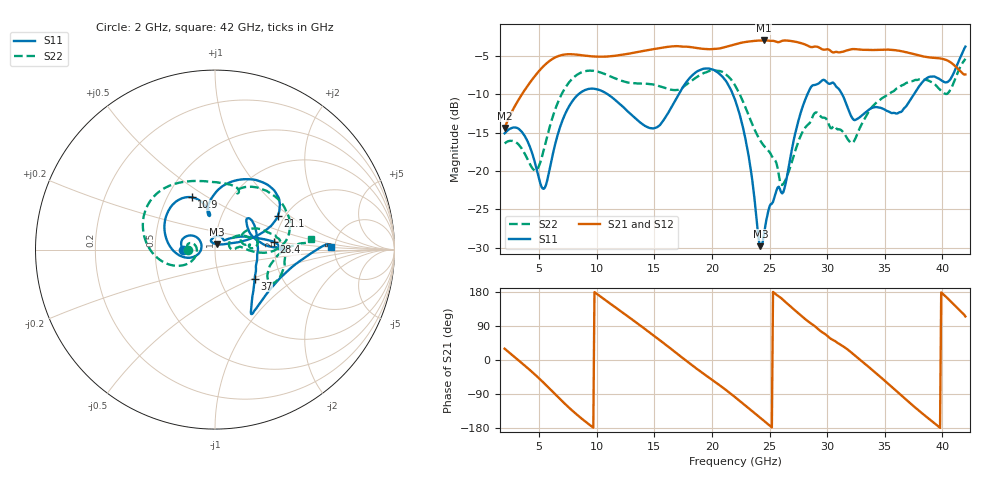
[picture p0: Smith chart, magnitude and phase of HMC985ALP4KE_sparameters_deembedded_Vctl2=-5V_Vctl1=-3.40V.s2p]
!s2p File: Measurements: S11, S21, S12, S22
# GHz S dB R 50.0
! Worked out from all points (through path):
!   401 points, 2 GHz to 42 GHz, reference 50 ohm
!   highest |S21| = -2.97 dB at 24.5 GHz (marker M1); lowest = -14.4 dB at 2 GHz (marker M2)
!   lowest |S11| = -29.8 dB at 24.2 GHz (marker M3), VSWR 1.07, Z = 50.8 + j3.16 ohm
!   |S11| at or under -10 dB: start of sweep to 8.403 GHz; 10.97 GHz to 17.11 GHz (6.144 GHz wide, 43.8 % of centre); 21.81 GHz to 28.29 GHz (6.471 GHz wide, 25.8 % of centre)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
!   |S22| runs from -21.8 to -5.4 dB; largest |S21 - S12| = 0.00075
!   S11 on the Smith chart (normalised r, x): 2 GHz: 0.70, -0.00; 10.9 GHz: 0.66, +0.43; 21.1 GHz: 1.84, +0.81; 28.4 GHz: 1.96, +0.19; 37 GHz: 1.46, -0.51; 42 GHz: 4.67, +0.19
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2  -15.08 -178.9  -14.38 29.8  -14.39 29.8  -16.39 -179.5
3.6  -15.10 155.1  -9.77 -10.9  -9.78 -10.9  -17.35 164.5
5.4  -22.31 174.3  -6.29 -60.3  -6.30 -60.3  -17.23 -154.6
6.9  -13.88 -171.0  -4.90 -105.7  -4.90 -105.7  -10.12 -169.4
8.7  -9.66 146.2  -4.90 -154.9  -4.90 -154.9  -7.12 153.5
10.9  -9.94 113.9  -5.07 154.7  -5.07 154.7  -7.47 118.4
13.4  -13.17 99.2  -4.52 99.5  -4.52 99.5  -8.55 84.5
15.4  -14.11 101.1  -3.99 53.9  -3.99 53.9  -8.92 68.5
17.9  -8.16 76.0  -3.80 -5.0  -3.80 -5.0  -8.60 67.0
21.1  -8.04 28.1  -3.85 -76.5  -3.86 -76.4  -7.27 15.7
22  -10.69 20.3  -3.48 -97.9  -3.48 -97.9  -8.82 2.1
23.1  -17.33 17.6  -3.13 -125.2  -3.13 -125.1  -12.41 -3.7
24.2  -29.78 73.2  -2.98 -152.5  -2.98 -152.5  -16.04 3.5
24.5  -28.34 106.3  -2.97 -160.1  -2.97 -160.1  -16.68 5.6
26.2  -22.73 44.9  -2.99 158.1  -2.99 158.1  -21.66 19.7
28.4  -9.61 7.6  -3.72 100.6  -3.72 100.7  -13.86 18.8
28.7  -8.86 2.6  -3.84 94.6  -3.85 94.6  -13.03 17.5
32.4  -13.36 27.1  -4.10 12.0  -4.10 12.0  -15.91 26.0
35.4  -12.28 13.9  -4.18 -65.5  -4.17 -65.5  -9.93 16.6
37  -11.24 -36.2  -4.56 -108.6  -4.56 -108.6  -8.45 3.6
39.7  -7.95 -54.9  -5.29 -176.5  -5.29 -176.5  -9.25 -30.6
42  -3.77 1.1  -7.40 115.0  -7.41 115.0  -5.36 6.3
